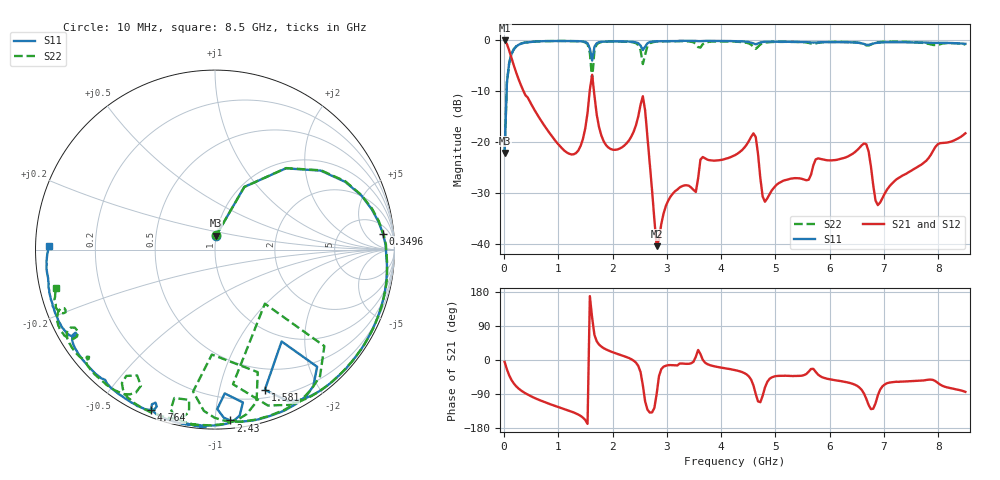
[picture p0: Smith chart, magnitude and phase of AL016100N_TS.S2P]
!AVX CORPORATION
!PART NUMBER AL016100N_TS
!DESCRIPTION: AIR CORE INDUCTOR, 100nH, 9 TURNS
!Agilent Technologies,E5071C,MY46102230,A.09.54
!Date: Mon Sep 03 16:38:55 2012
!Data & Calibration Information:
!Freq	S11:SOLT2(ON)	S21:SOLT2(ON)	S12:SOLT2(ON)	S22:SOLT2(ON)
# Hz S dB R 50
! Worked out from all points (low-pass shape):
!   201 points, 10 MHz to 8.5 GHz, reference 50 ohm
!   highest |S21| = -0.03 dB at 10 MHz (marker M1); lowest = -40.4 dB at 2.812 GHz (marker M2)
!   |S21| within 3 dB of the highest: start of sweep to 124.2 MHz
!   lowest |S11| = -22.1 dB at 10 MHz (marker M3), VSWR 1.17, Z = 50 + j7.88 ohm
!   |S11| at or under -10 dB: start of sweep to 47.16 MHz
!   |S22| runs from -22.0 to -0.1 dB; largest |S21 - S12| = 0.0069
!   S11 on the Smith chart (normalised r, x): 10 MHz: 1.00, +0.16; 349.6 MHz: 10, +15; 1.581 GHz: 0.28, -1.38; 2.43 GHz: 0.05, -1.09; 4.764 GHz: 0.03, -0.68; 8.5 GHz: 0.04, +0.01
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1e7  -22.09 85.3  -0.03 -4.9  -0.07 -5.2  -22.01 85.6
9.49e7  -4.43 48.9  -2.01 -40.7  -1.99 -40.7  -4.40 48.9
3.496e8  -0.54 5.4  -9.77 -84.0  -9.75 -84.0  -0.52 5.5
1.1137e9  -0.13 -40.3  -21.67 -129.6  -21.66 -129.7  -0.14 -41.4
1.4533e9  -0.23 -57.1  -19.36 -152.1  -19.35 -152.1  -0.28 -60.8
1.58065e9  -1.63 -70.4  -9.69 168.6  -9.69 168.6  -2.42 -82.4
1.6231e9  -3.98 -54.1  -6.76 111.1  -6.76 111.1  -7.75 -47.3
1.66555e9  -1.25 -48.9  -10.89 66.0  -10.89 65.9  -1.80 -41.4
1.92025e9  -0.21 -66.2  -21.02 25.2  -21.01 25.2  -0.24 -66.5
2.42965e9  -0.39 -84.9  -16.68 -6.9  -16.69 -6.9  -0.56 -90.1
2.557e9  -1.91 -86.1  -10.97 -66.6  -10.96 -66.7  -4.66 -91.7
2.8117e9  -0.19 -89.1  -40.39 -89.6  -40.30 -88.2  -0.24 -86.7
2.85415e9  -0.18 -90.2  -39.07 -42.7  -39.13 -42.1  -0.22 -88.5
3.6607e9  -0.13 -98.2  -22.89 0.6  -22.90 0.5  -0.76 -99.1
4.255e9  -0.16 -106.5  -22.53 -26.6  -22.53 -26.8  -0.28 -116.0
4.5946e9  -0.62 -112.2  -18.26 -66.9  -18.26 -66.9  -1.31 -125.1
4.7644e9  -0.33 -111.8  -30.63 -94.5  -30.71 -94.7  -0.57 -120.5
5.6983e9  -0.45 -130.1  -24.53 -23.4  -24.55 -23.9  -0.71 -139.6
6.6322e9  -0.71 -149.1  -20.24 -88.6  -20.22 -88.6  -0.79 -151.6
6.8869e9  -0.47 -150.5  -32.34 -93.3  -32.42 -93.2  -0.39 -149.1
7.09915e9  -0.37 -155.2  -28.68 -59.6  -28.75 -59.9  -0.26 -152.0
8.5e9  -0.68 178.8  -18.24 -84.1  -18.25 -84.0  -0.82 -166.3
